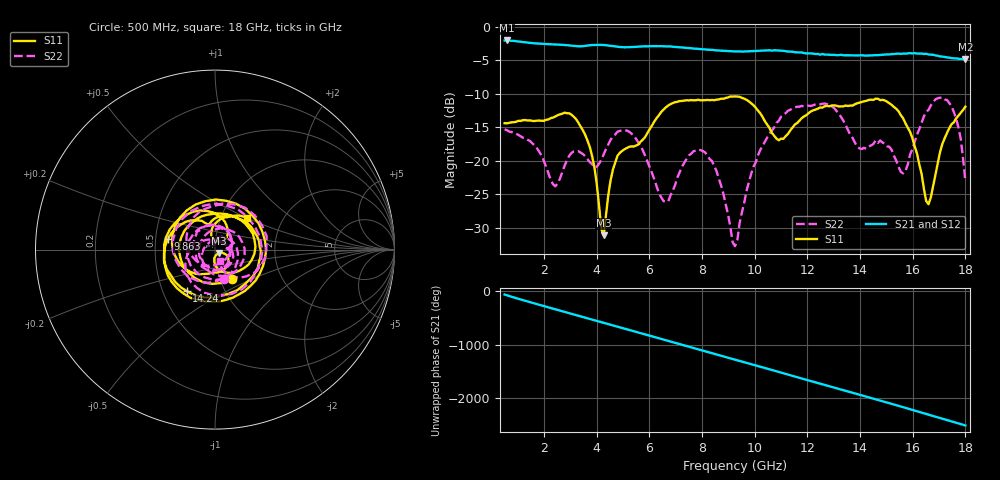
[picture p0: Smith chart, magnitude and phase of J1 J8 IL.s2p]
!Agilent Technologies,N5230A,MY45001360,A.07.50.67
!Agilent N5230A: A.07.50.67
!Date: Tuesday, April 16, 2024 16:36:35
!Correction: S11(Full 2 Port(1,2))
!S21(Full 2 Port(1,2))
!S12(Full 2 Port(1,2))
!S22(Full 2 Port(1,2))
!S2P File: Measurements: S11, S21, S12, S22:
# Hz S  dB  R 50
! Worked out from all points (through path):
!   201 points, 500 MHz to 18 GHz, reference 50 ohm
!   highest |S21| = -2.07 dB at 587.5 MHz (marker M1); lowest = -4.9 dB at 18 GHz (marker M2)
!   group delay of S21, straight-line fit = 388 ps
!   lowest |S11| = -31.1 dB at 4.263 GHz (marker M3), VSWR 1.06, Z = 52.1 - j1.97 ohm
!   |S11| at or under -10 dB: start of sweep to end of sweep
!   |S22| runs from -32.7 to -10.5 dB; largest |S21 - S12| = 0.009
!   S11 on the Smith chart (normalised r, x): 500 MHz: 1.14, -0.39; 9.863 GHz: 0.58, +0.07; 14.24 GHz: 0.66, -0.33; 18 GHz: 1.33, +0.51
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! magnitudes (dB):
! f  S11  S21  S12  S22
! 500 MHz  -14.4  -2.1  -2.1  -15.3
! 587.5 MHz  -14.4  -2.1  -2.1  -15.4
! 2.425 GHz  -13.4  -2.7  -2.7  -23.8
! 3.475 GHz  -15.5  -2.9  -2.9  -19.0
! 3.913 GHz  -21.0  -2.7  -2.7  -21.0
! 4.263 GHz  -31.1  -2.8  -2.7  -19.0
! 4.787 GHz  -19.2  -3.0  -3.0  -15.7
! 5.487 GHz  -17.7  -3.0  -3.0  -16.7
! 6.362 GHz  -13.2  -2.9  -2.9  -24.8
! 8.113 GHz  -11.0  -3.4  -3.4  -18.7
! 8.55 GHz  -10.9  -3.6  -3.5  -21.5
! 9.25 GHz  -10.4  -3.7  -3.7  -32.7
! 9.863 GHz  -11.4  -3.7  -3.7  -22.0
! 10.91 GHz  -16.9  -3.6  -3.6  -14.0
! 12.22 GHz  -12.5  -4.0  -4.0  -11.7
! 14.24 GHz  -11.1  -4.3  -4.3  -18.2
! 15.11 GHz  -11.4  -4.1  -4.1  -17.9
! 15.64 GHz  -13.7  -4.0  -4.0  -21.9
! 16.6 GHz  -26.5  -4.2  -4.2  -12.4
! 17.48 GHz  -14.5  -4.7  -4.6  -11.9
! 17.82 GHz  -12.8  -4.8  -4.8  -16.8
! 18 GHz  -11.9  -4.9  -4.9  -23.1
